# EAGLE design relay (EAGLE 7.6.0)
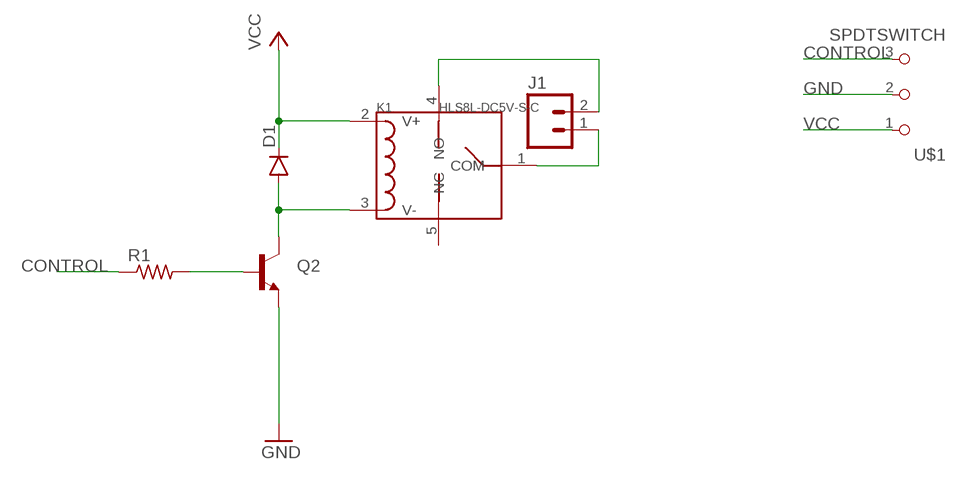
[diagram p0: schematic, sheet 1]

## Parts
D1  DIODEPTH  [DIODE-1N4001]
J1  M02POLAR_LOCK  [MOLEX-1X2_LOCK]
K1  HLS8L-DC5V-S-C  RELAY-HLS8L-DC5V-S-C(5P-19X15MM)  [REY5-19.0X15.0X15.0MM]
Q2  TRANSISTOR_NPNBC547  [TO-92-AMMO]
R1  RES-US1206FAB  [R1206FAB]
U$1  SPDTSWITCH  [SPDTSWITCH]

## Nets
CONTROL: R1.1 U$1.3
GND: Q2.3(E) U$1.2
N$1: J1.2 K1.4(NO)
N$2: D1.A K1.3(V-) Q2.1(C)
N$3: Q2.2(B) R1.2
N$4: J1.1 K1.1(COM)
VCC: D1.C K1.2(V+) U$1.1
Unconnected: K1.5(NC)

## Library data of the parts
D1 = SparkFun-DiscreteSemi:DIODE: Diode
J1 = SparkFun-Connectors:M02: Standard 2-pin 0.1" header. Use with
K1 = Seeed-OPL-Relay:RELAY-HLS8L-DC5V-S-C(5P-19X15MM): 315030000; MPN: HLS8L-DC5V-S-C
Q2 = SparkFun-DiscreteSemi:TRANSISTOR_NPN: Generic NPN BJT MMBT2222A - TRANS-08049 (SOT-23, 1A 40V) MPSA42 - TRANS-09116 (SOT-23, 500mA 300V) MMBT5088LT1G - TRANS-11160 (SOT-23, 50 mA 30V) BC547 - COM-08928 (TO-92 45V 100mA) (1.Collector 2.Base 3.Emitter) 2N3904 - COM-00521 (TO-92 40V 200mA) (1.Emitter 2.Base 3.Collector) P2N2222A -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
R1 = fab:RES-US: Resistor (US Symbol)
U$1 = fab:SPDTSWITCH

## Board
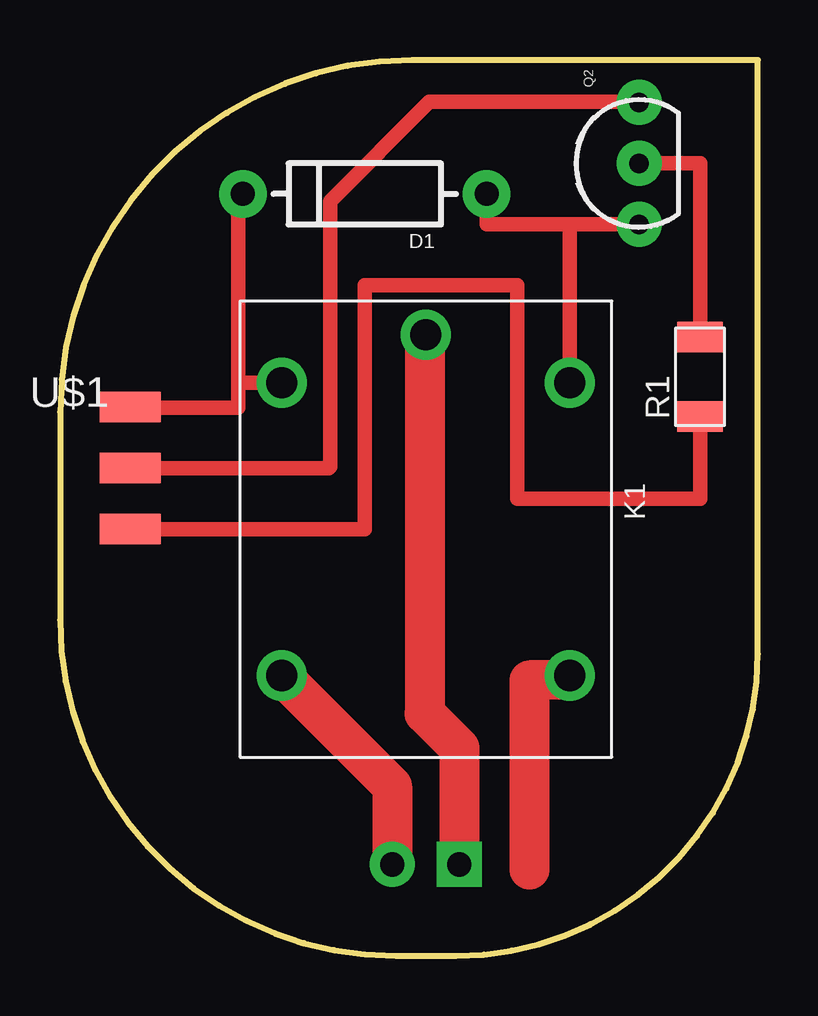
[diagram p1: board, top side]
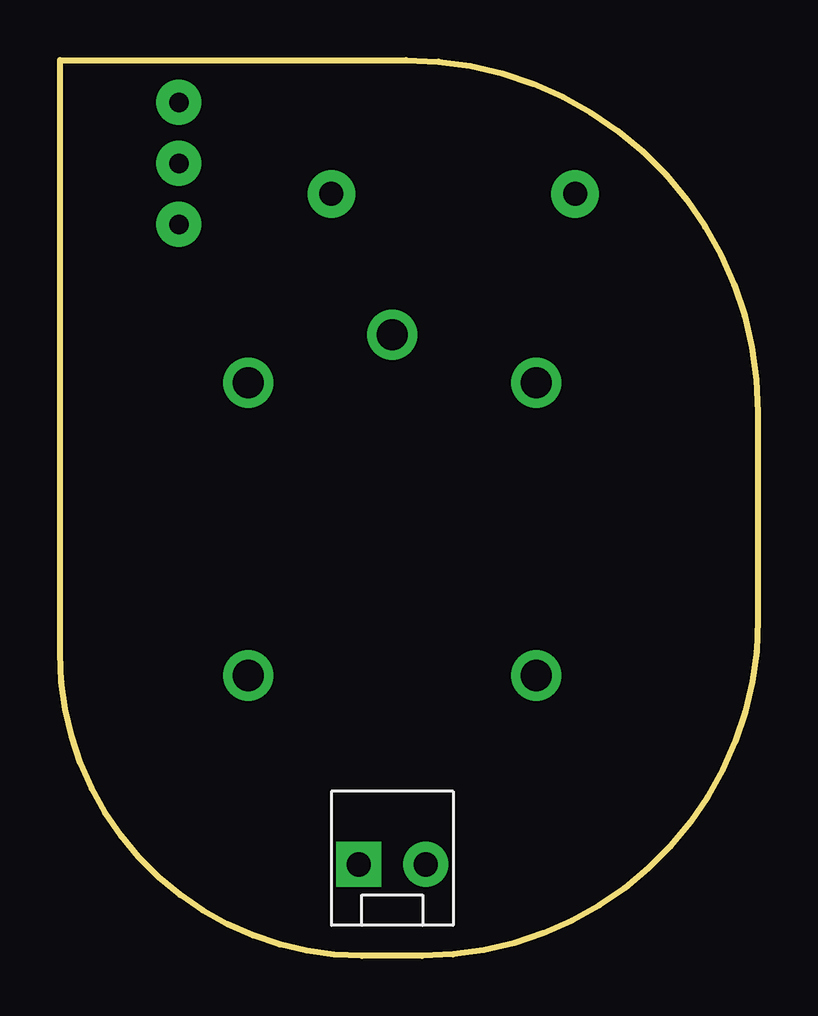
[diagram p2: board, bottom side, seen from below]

Size 29.08 x 37.33 mm. Coordinates in mm from the lower left corner, seen from the top.
Outline: 29.08,37.33 14.68,37.33 arc90 0,22.65 0,13.99 arc90 13.99,0 16.5,0 arc90 29.08,12.59 29.08,37.33
Copper layers (1*16): Top 0.035mm / dielectric 1.5mm / Bottom 0.035mm
Design rules "default": minimum track width 10mil, minimum drill 24mil, track to track 8mil, track to pad 8mil, pad to pad 8mil, via to via 8mil, smd to smd 8mil, copper to edge 40mil, drill to drill 8mil, minimum pad ring 10mil, minimum via ring 8mil, stop-mask expansion 4mil, vias tented up to drill 0mil, thermal gap 10mil

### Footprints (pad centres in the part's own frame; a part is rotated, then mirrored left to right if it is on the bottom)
DIODE-1N4001 = drill 1 pad 1.981: A -5.08,0; C 5.08,0
MOLEX-1X2_LOCK = drill 1.016 pad 1.88 square: 1 -0.127,0 | drill 1.016 pad 1.88: 2 2.667,0
REY5-19.0X15.0X15.0MM = drill 1.3 pad 2.1: 1 -8.1,0; 2 -6.1,-6; 3 -6.1,6; 4 6.1,-6; 5 6.1,6
TO-92-AMMO = drill 0.813 pad 1.88: 1 -2.54,0; 2 0,0; 3 2.54,0
R1206FAB = smd 1.27 x 1.905: 1 -1.651,0; 2 1.651,0
SPDTSWITCH = smd 2.54 x 1.27: 1 0.38,2.54; 2 0.38,0; 3 0.38,-2.54

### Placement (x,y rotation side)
D1  12.7,31.75 180 top
J1  16.51,3.81 0 bottom
K1  15.24,17.78 270 top
Q2  24.13,33.02 90 top
R1  26.67,24.13 90 top
U$1  2.54,20.32 0 top

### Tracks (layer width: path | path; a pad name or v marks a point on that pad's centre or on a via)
CONTROL
  Top 0.406: U$1.3 3.81,17.78
  Top 0.61: R1.1 26.67,19.05 19.05,19.05 19.05,27.94 12.7,27.94 12.7,17.78 3.81,17.78
GND
  Top 0.61: Q2.3 24.11,35.59 15.39,35.59 11.25,31.45 11.25,20.37 11.2,20.32 U$1.2
N$1
  Top 1.676: K1.4 13.84,7.08 J1.2
N$2
  Top 0.61: D1.A 17.78,30.48 21.24,30.48 | 21.24,30.48 K1.3 | Q2.1 21.24,30.48
N$3
  Top 0.61: Q2.2 26.67,33.02 R1.2
N$4
  Top 1.676: K1.1 15.19,25.88 15.19,10.11 16.64,8.66 J1.1
N$5
  Top 1.676: 21.23,11.51 19.56,11.48 19.56,3.61
VCC
  Top 0.61: K1.2 7.42,23.88 | D1.C 7.42,31.75 7.42,23.88 | 7.42,23.88 7.42,22.84 2.92,22.84 U$1.1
